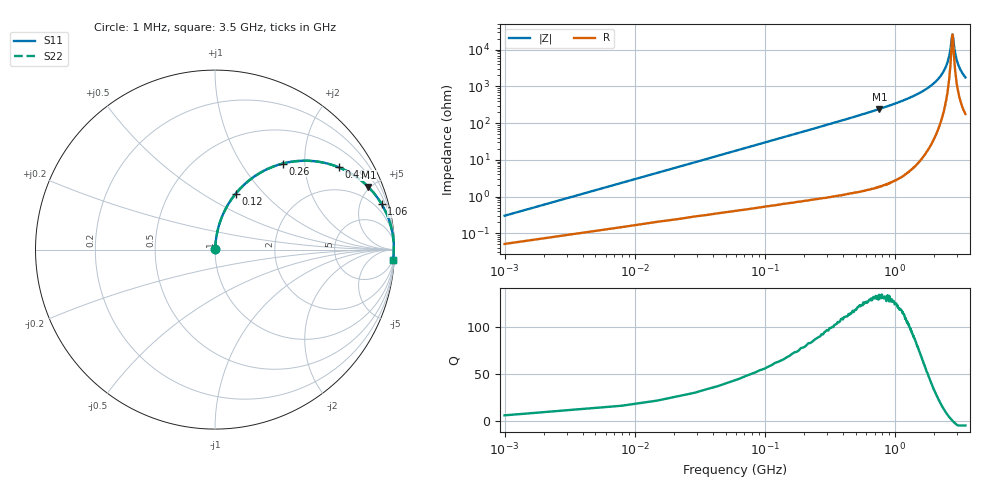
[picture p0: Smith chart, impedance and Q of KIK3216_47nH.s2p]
!version-2
!date-01.2022
!Series
# MHz S RI R 50
!Freq ReS11 ImS11 ReS21 ImS21 ReS12 ImS12 ReS22 ImS22
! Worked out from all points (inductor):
!   501 points, 1 MHz to 3.5 GHz, reference 50 ohm
!   read as one part in series: L = 47 nH near 15 MHz
!   highest Q = 132 at 764 MHz (marker M1), where L = 50.8 nH
!   self-resonance near 2.78 GHz
!   S11 on the Smith chart (normalised r, x): 1 MHz: 1.00, +0.01; 120 MHz: 1.01, +0.71; 260 MHz: 1.02, +1.55; 491 MHz: 1.03, +2.99; 1.06 GHz: 1.06, +7.31; 3.5 GHz: 5, -35
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1  0.000538 0.00295  0.9995 -0.00295  0.9995 -0.00295  0.000538 0.00295
22  0.00664 0.0644  0.9934 -0.0644  0.9934 -0.0644  0.00664 0.0644
36  0.0142 0.1045  0.9858 -0.1045  0.9858 -0.1045  0.0142 0.1045
71  0.0461 0.1993  0.954 -0.1993  0.954 -0.1993  0.0461 0.1993
120  0.1159 0.3121  0.8841 -0.3121  0.8841 -0.3121  0.1159 0.3121
260  0.3763 0.4789  0.6237 -0.4789  0.6237 -0.4789  0.3763 0.4789
491  0.6899 0.4583  0.3101 -0.4583  0.3101 -0.4583  0.6899 0.4583
589  0.7665 0.4191  0.2335 -0.4191  0.2335 -0.4191  0.7665 0.4191
764  0.8543 0.349  0.1457 -0.349  0.1457 -0.349  0.8543 0.349
1060  0.9285 0.2536  0.0715 -0.2536  0.0715 -0.2536  0.9285 0.2536
1170  0.9445 0.2246  0.0555 -0.2246  0.0555 -0.2246  0.9445 0.2246
1760  0.9847 0.1137  0.0153 -0.1137  0.0153 -0.1137  0.9847 0.1137
2340  0.9953 0.0422  0.00472 -0.0422  0.00472 -0.0422  0.9953 0.0422
2490  0.9961 0.0274  0.00394 -0.0274  0.00394 -0.0274  0.9961 0.0274
2630  0.9963 0.0141  0.00366 -0.0141  0.00366 -0.0141  0.9963 0.0141
2780  0.9962 0.000314  0.00379 -0.000314  0.00379 -0.000314  0.9962 0.000314
2820  0.9961 -0.0027  0.00387 0.0027  0.00387 0.0027  0.9961 -0.0027
2870  0.996 -0.00745  0.00405 0.00745  0.00405 0.00745  0.996 -0.00745
2920  0.9958 -0.0115  0.00424 0.0115  0.00424 0.0115  0.9958 -0.0115
3000  0.9954 -0.0184  0.00465 0.0184  0.00465 0.0184  0.9954 -0.0184
3150  0.9944 -0.0299  0.00557 0.0299  0.00557 0.0299  0.9944 -0.0299
3500  0.9913 -0.0553  0.00872 0.0553  0.00872 0.0553  0.9913 -0.0553
